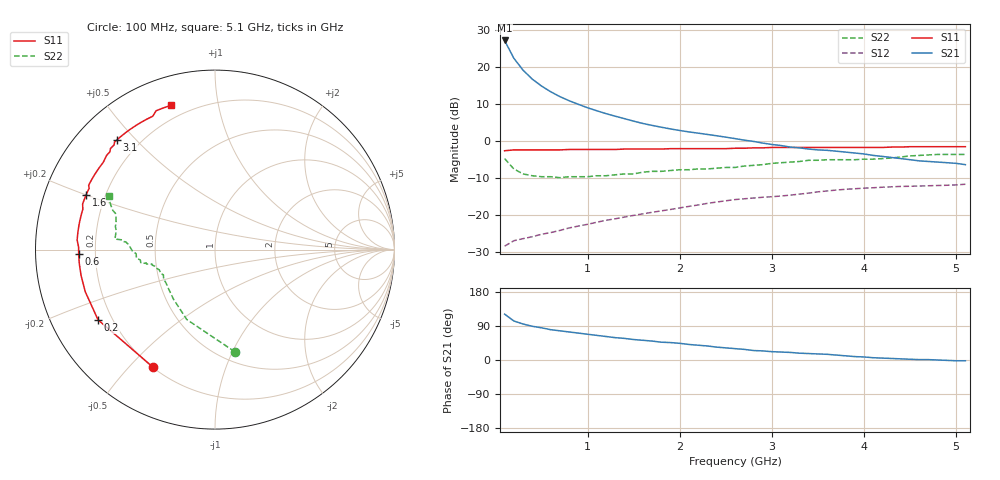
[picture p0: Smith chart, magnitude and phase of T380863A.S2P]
!AT-38086
!S-PARAMETERS at Vce=3.6V  Ic=30mA.  LAST UPDATED 08-05-96
# ghz s ma r 50
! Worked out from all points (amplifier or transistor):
!   51 points, 100 MHz to 5.1 GHz, reference 50 ohm
!   highest |S21| = 27.2 dB at 100 MHz (marker M1)
!   |S21| within 3 dB of that: start of sweep to 162.4 MHz
!   unconditionally stable (mu >= 1): 934.5 MHz to end of sweep
!   at 900 MHz: K = 0.98, MSG = 16.5 dB, |S12| = -23.0 dB
!   at 2.6 GHz: K = 1.10, MAG = 6.3 dB, |S12| = -15.8 dB
!   at 5.1 GHz: K = 1.10, MAG = 0.7 dB, |S12| = -11.7 dB
!   S11 on the Smith chart (normalised r, x): 100 MHz: 0.20, -0.58; 200 MHz: 0.15, -0.27; 600 MHz: 0.14, -0.02; 1.6 GHz: 0.13, +0.20; 3.1 GHz: 0.12, +0.44; 5.1 GHz: 0.13, +0.73
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0.1  0.74 -118.0  22.9 121.0  0.038 40.0  0.58 -79.0
0.2  0.76 -149.0  13.17 103.0  0.045 32.0  0.42 -112.0
0.3  0.76 -162.0  9.09 95.0  0.048 32.0  0.36 -130.0
0.4  0.76 -169.0  6.88 89.0  0.051 34.0  0.34 -139.0
0.5  0.76 -174.0  5.55 85.0  0.055 37.0  0.33 -146.0
0.6  0.76 -178.0  4.64 80.0  0.058 40.0  0.33 -150.0
0.7  0.76 179.0  3.99 77.0  0.062 42.0  0.32 -154.0
0.8  0.77 176.0  3.51 74.0  0.067 45.0  0.33 -156.0
0.9  0.77 173.0  3.14 71.0  0.071 46.0  0.33 -159.0
1  0.77 170.0  2.82 68.0  0.075 48.0  0.33 -160.0
1.2  0.77 165.0  2.35 62.0  0.085 51.0  0.34 -163.0
1.3  0.77 163.0  2.17 59.0  0.089 52.0  0.35 -165.0
1.6  0.78 157.0  1.73 52.0  0.104 54.0  0.38 -168.0
1.8  0.78 154.0  1.54 47.0  0.114 55.0  0.39 -169.0
2.1  0.79 150.0  1.33 41.0  0.131 56.0  0.41 -170.0
2.6  0.8 139.0  1.08 30.0  0.162 54.0  0.44 -177.0
2.8  0.81 136.0  0.99 25.0  0.17 52.0  0.47 179.0
3.1  0.82 132.0  0.87 21.0  0.181 51.0  0.51 175.0
3.5  0.82 128.0  0.76 16.0  0.206 50.0  0.55 174.0
4.3  0.83 114.0  0.6 4.0  0.241 41.0  0.59 160.0
4.8  0.84 110.0  0.52 0.0  0.251 36.0  0.66 154.0
5.1  0.84 107.0  0.48 -2.0  0.261 35.0  0.66 153.0
